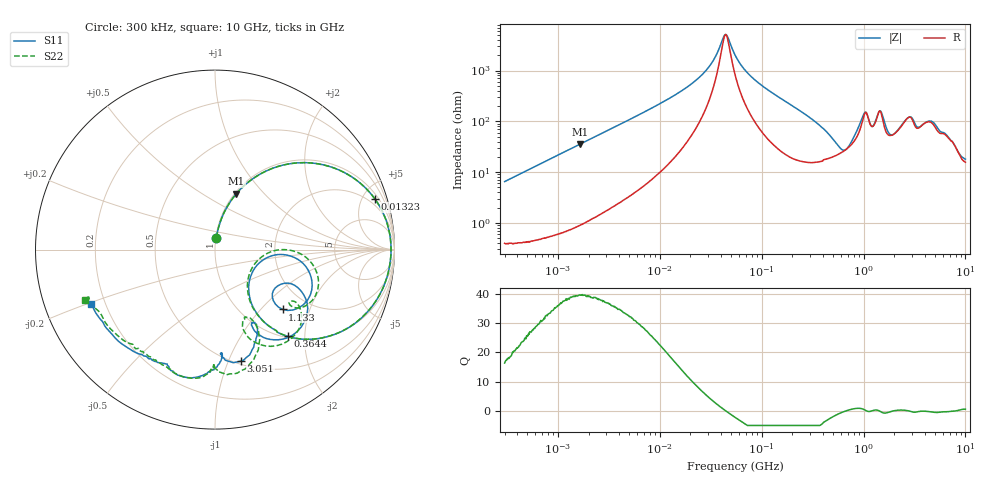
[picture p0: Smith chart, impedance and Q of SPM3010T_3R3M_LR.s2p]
! S-Parameter Data Generated by TDK Corporation
! Copyright(C) 2019 TDK Corporation.
! All Rights Reserved.
! TDK P/N: SPM3010T-3R3M-LR (Inductor)
! Property: L=3.3uH at 100kHz
! Size(LxWxT): 3.2x3x1mm
! Model Type: s2p (Touchstone File Format Version 1.0)
! Frequency: DC=Yes Start=0.3MHz Stop=10000MHz 802points Log-sweep
! Model Generated on Sep. 23, 2019
! Port Assignments:
!  1 ---@@@--- 2
! Applicable Conditions:
!  Temperature = 25 degC
!  DC Bias Current = 0 A
!  Small Signal Operation
! Terms and conditions regarding TDK Simulation Models
! (1)This simulation model is being provided solely for informational purposes. Please refer to the specifications of the products in terms of detailed characteristics of such products.
! (2)In no event shall TDK Corporation of any of its subsidiaries be liable for any loss or damage arising, directly or indirectly,
!  From any information contained in this simulation model, including, but not limited to loss or damages arising from any inaccuracies, omissions or errors in connection with such information.
! (3)Any and all copyrights on this simulation model are owned by TDK Corporation.
!  Duplication or redistribution of this simulation model without prior written permission from TDK Corporation is prohibited.
! (4)This simulation model is subject to any modification or change without any prior notice.
! (5)Neither TDK Corporation nor any of its subsidiaries shall make any warranty, express or implied,
!  Including but not limited to the correctness, implied warranties of merchantability and fitness for a particular purpose with respect to this simulation models.
! (6)The use of this simulation model shall be deemed to have consented to the terms and conditions hereof.
# Hz S MA R 50
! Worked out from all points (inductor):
!   801 points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, 300 kHz to 10 GHz, reference 50 ohm
!   read as one part in series: L = 3.43 uH near 318.3 kHz
!   highest Q = 39.6 at 1.667 MHz (marker M1), where L = 3.42 uH
!   self-resonance near 44.4 MHz
!   S11 on the Smith chart (normalised r, x): 300 kHz: 1.01, +0.13; 13.23 MHz: 1.38, +6.18; 364.4 MHz: 1.02, -1.65; 1.133 GHz: 1.50, -1.34; 3.051 GHz: 0.53, -1.11; 10 GHz: 0.15, -0.21
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300000  0.06595 83.1  0.9936 -3.6  0.9935 -3.6  0.06573 83.3
1666935  0.3345 69.0  0.9339 -19.5  0.9341 -19.5  0.3345 69.0
1713600  0.3427 68.5  0.9308 -20.0  0.9309 -20.0  0.3426 68.5
4363314  0.6726 46.0  0.7202 -42.3  0.7204 -42.3  0.6726 46.0
9671944  0.8909 24.4  0.4172 -63.1  0.4175 -63.1  0.8907 24.4
1.322782e7  0.9348 17.5  0.3066 -69.2  0.3068 -69.2  0.9346 17.5
2.725275e7  0.9767 5.5  0.1073 -75.1  0.1073 -75.1  0.9765 5.5
4.38171e7  0.9809 -0.8  0.01925 -9.1  0.01926 -9.1  0.9807 -0.8
5.477226e7  0.979 -3.8  0.0482 61.9  0.04823 61.9  0.9789 -3.8
1.050124e8  0.9568 -13.9  0.2006 69.5  0.2007 69.5  0.9565 -13.8
3.126428e8  0.713 -44.6  0.6126 37.8  0.6128 37.8  0.7113 -44.6
3.644326e8  0.6308 -50.0  0.6751 30.1  0.6753 30.1  0.6287 -50.1
6.987102e8  0.2431 -28.4  0.7632 -12.0  0.7634 -12.1  0.2306 -27.7
9.101824e8  0.447 -5.8  0.5822 -34.0  0.5824 -34.0  0.4374 -1.0
1.133369e9  0.5032 -41.5  0.4645 -12.7  0.4647 -12.7  0.5758 -34.2
1.307877e9  0.448 -24.7  0.4845 -30.8  0.4847 -30.8  0.5398 -33.1
1.43752e9  0.6124 -32.4  0.3539 -24.5  0.3541 -24.5  0.6432 -43.2
1.767019e9  0.5207 -63.3  0.5628 -18.2  0.563 -18.2  0.4816 -70.4
2.23379e9  0.4749 -61.0  0.5132 -42.7  0.5137 -42.7  0.4411 -62.2
3.050901e9  0.6384 -77.1  0.3583 -37.7  0.3585 -37.7  0.7003 -81.2
5.157474e9  0.7301 -103.1  0.3247 -50.9  0.3246 -51.0  0.7291 -106.4
1e10  0.7518 -156.3  0.2853 -96.6  0.2858 -96.7  0.7786 -158.9
